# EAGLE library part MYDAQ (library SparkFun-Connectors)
myDAQ This connecotr is used in the National Instruments myDAQ measurement and control tool ecosystem. Learn more at the myDAQ website. The connector is a 20pin 3.81mm spaced Female Right Angle Terminal Block (PTH). Sorry, we do not sell the connector as an individual part at SparkFun, howere here is a link to the datasheet: Datasheet It is used on this SparkFun product: SparkFun myDAQ Protoboard Kit (DEV-10705)
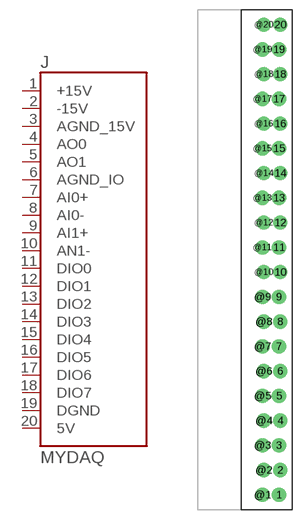
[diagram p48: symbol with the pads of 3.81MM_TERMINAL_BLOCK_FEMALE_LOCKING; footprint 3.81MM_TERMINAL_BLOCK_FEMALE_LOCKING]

Designator prefix J

## MYDAQ (PROD_ID: CONN-10450)  [3.81MM_TERMINAL_BLOCK_FEMALE_LOCKING]
1  +15V  pwr
2  -15V  pwr
3  AGND_15V  pwr
4  AO0  out
5  AO1  out
6  AGND_IO  pwr
7  AI0+  in
8  AI0-  in
9  AI1+  in
10  AN1-  in
11  DIO0
12  DIO1
13  DIO2
14  DIO3
15  DIO4
16  DIO5
17  DIO6
18  DIO7
19  DGND  pwr
20  5V  pwr

## Footprint 3.81MM_TERMINAL_BLOCK_FEMALE_LOCKING (pad centres in mm)
MyDAQ Female Right Angle Terminal Block w/ Locking Footprint Specifications: Pin count: 40 Pin pitch:3.18mm Datasheet referenced for footprint Example device(s): MyDAQ
drill 1.2 pad 2.184: 1 4.521,-36.194; 2 4.724,-32.384; 3 4.521,-28.574; 4 4.724,-24.764; 5 4.521,-20.954; 6 4.724,-17.144; 7 4.521,-13.334; 8 4.724,-9.524; 9 4.521,-5.714; 10 4.724,-1.904; 11 4.521,1.906; 12 4.724,5.716; 13 4.521,9.526; 14 4.724,13.336; 15 4.521,17.146; 16 4.724,20.956; 17 4.521,24.766; 18 4.724,28.576; 19 4.521,32.386; 20 4.724,36.196; @1 1.981,-36.194; @2 2.184,-32.384; @3 1.981,-28.574; @4 2.184,-24.764; @5 1.981,-20.954; @6 2.184,-17.144; @7 1.981,-13.334; @8 2.184,-9.524; @9 1.981,-5.714; @10 2.184,-1.904; @11 1.981,1.906; @12 2.184,5.716; @13 1.981,9.526; @14 2.184,13.336; @15 1.981,17.146; @16 2.184,20.956; @17 1.981,24.766; @18 2.184,28.576; @19 1.981,32.386; @20 2.184,36.196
